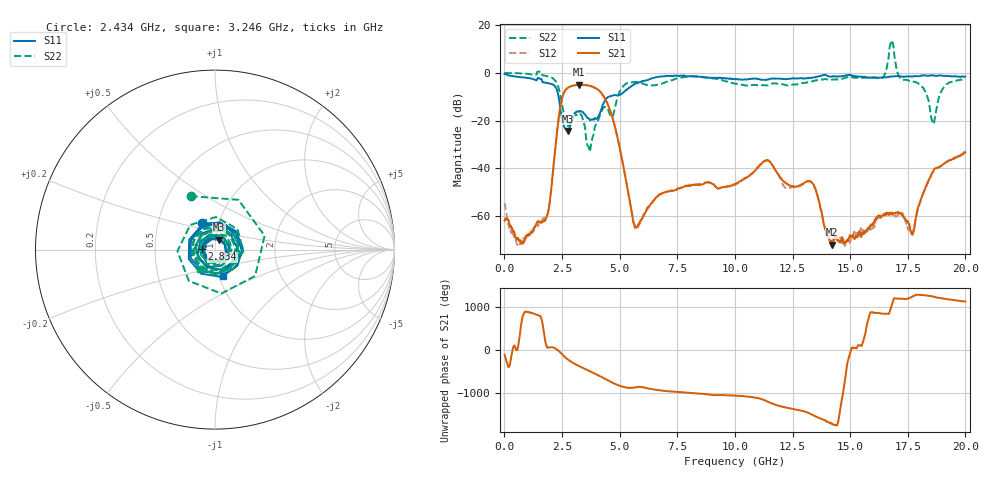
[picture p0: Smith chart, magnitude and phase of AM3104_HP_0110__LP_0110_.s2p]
!Created with skrf (http://scikit-rf.org).
# Hz S RI R 50.0
!freq ReS11 ImS11 ReS21 ImS21 ReS12 ImS12 ReS22 ImS22
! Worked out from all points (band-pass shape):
!   1601 points, 10 MHz to 20 GHz, reference 50 ohm
!   highest |S21| = -4.99 dB at 3.246 GHz (marker M1); lowest = -72.1 dB at 14.23 GHz (marker M2)
!   |S21| within 3 dB of the highest: 2.602 GHz to 4.171 GHz (1.569 GHz wide, 46.3 % of centre)
!   lowest |S11| = -24.4 dB at 2.759 GHz (marker M3), VSWR 1.13, Z = 52.1 + j5.77 ohm
!   |S11| at or under -10 dB: 2.352 GHz to 4.521 GHz (2.169 GHz wide, 63.1 % of centre)
!   |S22| runs from -33.1 to 13.6 dB; largest |S21 - S12| = 0.03
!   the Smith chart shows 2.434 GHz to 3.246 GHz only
!   S11 on the Smith chart (normalised r, x): 2.434 GHz: 0.83, +0.25; 2.834 GHz: 0.87, +0.00; 3.246 GHz: 1.05, -0.31
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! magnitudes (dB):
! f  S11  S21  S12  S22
! 10 MHz  -0.4  -62.0  -54.6  0.0
! 609.7 MHz  -1.7  -69.6  -72.3  -0.1
! 1.809 GHz  -4.1  -61.1  -60.2  -1.2
! 2.434 GHz  -15.5  -13.9  -13.9  -9.7
! 2.759 GHz  -24.4  -6.2  -6.2  -22.3
! 2.834 GHz  -22.8  -5.8  -5.8  -21.5
! 3.246 GHz  -16.3  -5.0  -5.1  -17.4
! 3.346 GHz  -16.2  -5.0  -5.1  -17.8
! 3.683 GHz  -19.4  -5.4  -5.4  -32.1
! 4.545 GHz  -9.9  -14.6  -14.7  -16.7
! 5.682 GHz  -4.5  -65.1  -64.5  -3.8
! 6.682 GHz  -1.6  -51.4  -51.6  -4.9
! 10.01 GHz  -2.7  -46.8  -46.9  -4.5
! 11.38 GHz  -2.9  -36.6  -36.8  -5.2
! 13.34 GHz  -2.1  -46.1  -46.0  -3.6
! 14.23 GHz  -1.5  -72.1  -70.9  -2.8
! 16.36 GHz  -1.9  -60.2  -59.9  -2.2
! 16.68 GHz  -1.6  -59.5  -59.3  7.2
! 17.7 GHz  -1.5  -68.0  -66.8  -3.7
! 18.6 GHz  -1.1  -41.4  -41.6  -21.4
! 19.09 GHz  -1.3  -38.0  -37.9  -5.7
! 20 GHz  -1.5  -33.4  -33.0  -2.5
